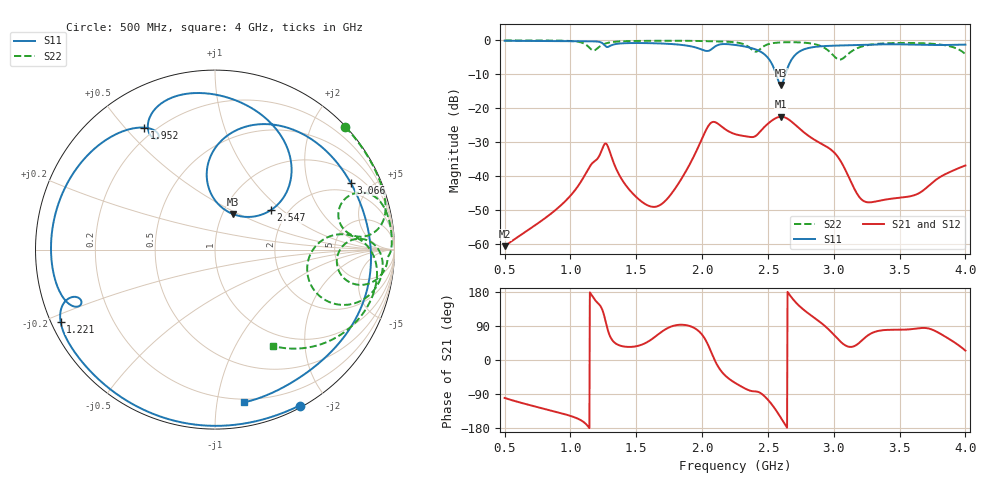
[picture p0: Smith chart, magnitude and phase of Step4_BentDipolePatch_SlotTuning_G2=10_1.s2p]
! TOUCHSTONE file generated by CST MICROWAVE STUDIO
! Date and time: Wed May 20 10:45:47 2020
! Project name: DualBand_DualMode_Antenna_FD_SteppedDesign.cst
! Parameters = {FPL=20; FPW=20; L=50; ST=10; SW=30; W=52; WF=7; ext=10; gap=1; inset=13}
! Header version: 2015
! Port assignment regex: !\s*Touchstone port\s*([0-9]+)\s*=\s*CST MWS port\s*([0-9]+)\s*\(\"(.*)\"\)(\s*mode\s*([0-9]+))?.*
! Touchstone port assignment:
! Touchstone port 1 = CST MWS port 1 ("")
! Touchstone port 2 = CST MWS port 2 ("")
# GHz S MA R 50
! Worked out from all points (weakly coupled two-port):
!   1006 points, 500 MHz to 4 GHz, reference 50 ohm
!   highest |S21| = -22.47 dB at 2.6 GHz (marker M1); lowest = -60.6 dB at 500 MHz (marker M2)
!   lowest |S11| = -13.1 dB at 2.596 GHz (marker M3), VSWR 1.57, Z = 55.8 + j23.3 ohm
!   |S11| at or under -10 dB: 2.563 GHz to 2.633 GHz (69.98 MHz wide, 2.69 % of centre)
!   |S22| runs from -5.7 to 0.0 dB; largest |S21 - S12| = 0.00024
!   S11 on the Smith chart (normalised r, x): 500 MHz: 0.02, -1.68; 1.221 GHz: 0.03, -0.22; 1.952 GHz: 0.16, +0.57; 2.547 GHz: 1.63, +0.84; 3.066 GHz: 1.46, +3.75; 4 GHz: 0.18, -1.20
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0.5  0.9886 -61.6  0.000937 -100.1  0.000937 -100.1  0.9968 43.3
0.794  0.9811 -97.8  0.002316 -128.3  0.002315 -128.2  0.9956 24.2
1.0845  0.9705 -134.3  0.008617 -160.0  0.008618 -160.0  0.9281 8.0
1.221  0.9494 -155.0  0.02033 145.5  0.02033 145.5  0.8093 21.9
1.2735  0.8025 -160.2  0.02993 92.8  0.02994 92.8  0.9075 20.2
1.452  0.9124 -175.8  0.006193 34.5  0.006195 34.5  0.9772 12.3
1.669  0.9027 156.5  0.003673 68.3  0.003672 68.3  0.9864 6.7
1.9525  0.785 120.1  0.02261 82.0  0.02261 82.0  0.9817 0.2
2.075  0.7497 119.4  0.06241 16.2  0.06241 16.2  0.9634 -2.6
2.25  0.8571 87.6  0.04178 -60.3  0.04177 -60.3  0.9371 -8.6
2.404  0.7394 60.9  0.03888 -82.8  0.03888 -82.8  0.6821 -5.8
2.5475  0.3804 35.3  0.06956 -125.6  0.06954 -125.6  0.9162 -0.6
2.5965  0.2216 63.7  0.07518 -151.5  0.07517 -151.5  0.9328 -3.3
2.6  0.2216 68.0  0.07523 -153.5  0.07521 -153.5  0.9336 -3.5
2.677  0.5106 93.2  0.06426 166.2  0.06427 166.2  0.94 -7.3
2.8345  0.7899 59.3  0.03636 116.0  0.03635 116.0  0.8964 -16.4
2.9605  0.8302 39.8  0.02618 80.9  0.02617 80.9  0.7026 -24.6
3.0655  0.8425 26.3  0.01511 44.1  0.01511 44.1  0.5362 -1.8
3.2195  0.8593 8.2  0.004425 53.4  0.004427 53.4  0.8186 3.4
3.419  0.8762 -15.0  0.004627 79.6  0.004634 79.7  0.9092 -7.2
3.7865  0.8547 -54.9  0.00918 73.8  0.00934 73.6  0.8778 -28.2
4  0.8661 -79.1  0.01441 24.8  0.01441 24.8  0.6247 -59.1
